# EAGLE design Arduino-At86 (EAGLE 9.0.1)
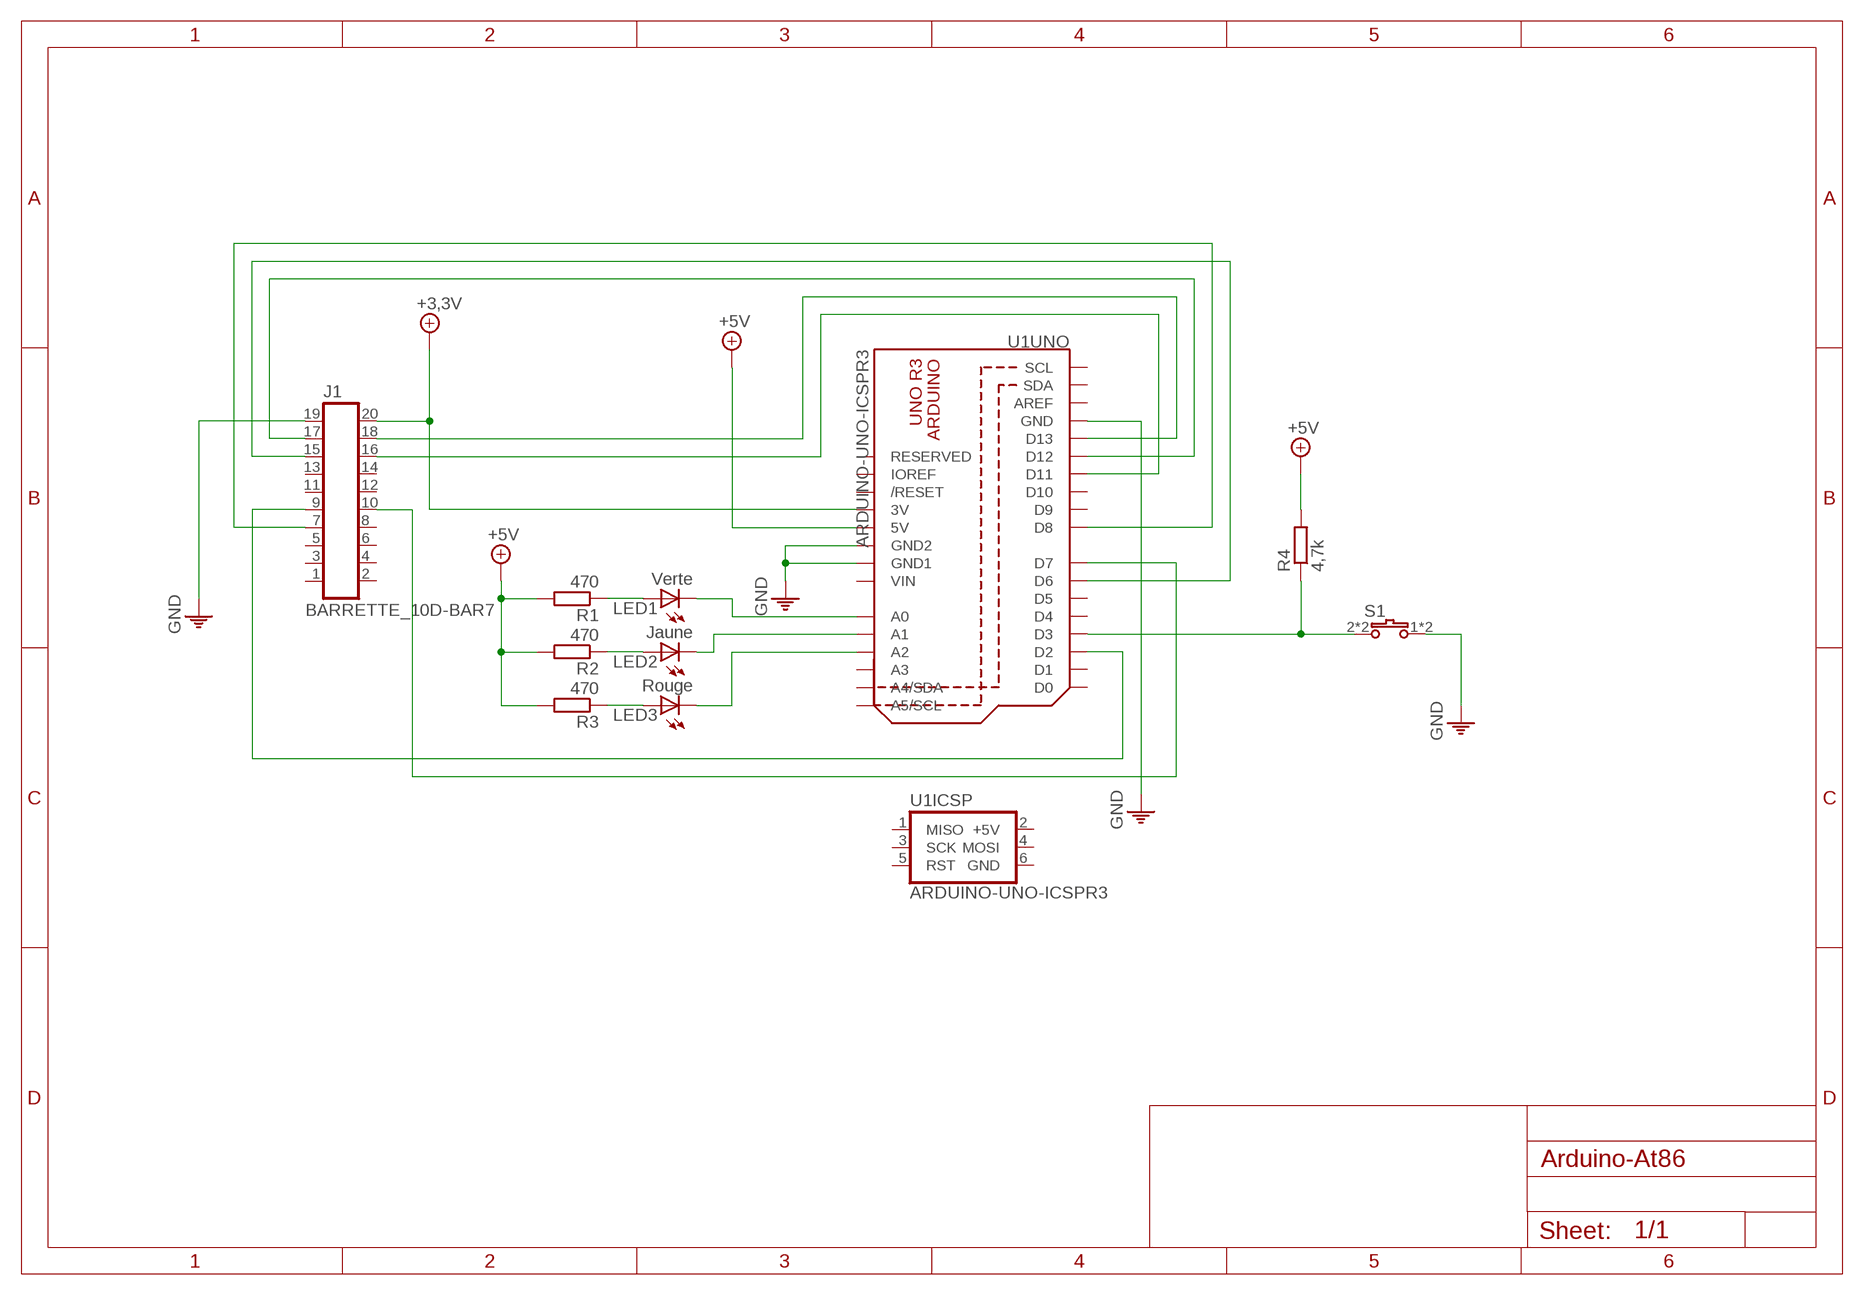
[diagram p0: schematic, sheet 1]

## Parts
J1  BARRETTE_10D-BAR7  [MA010-D]
LED1  Verte  LED3MM  [LED3MM]
LED2  Jaune  LED3MM  [LED3MM]
LED3  Rouge  LED3MM  [LED3MM]
R1  470  RCMS1206  [RCMS1206]
R2  470  RCMS1206  [RCMS1206]
R3  470  RCMS1206  [RCMS1206]
R4  4,7k  RCMS1206  [RCMS1206]
S1  BP-KSA  [TL1105]
U1  ARDUINO-UNO-ICSPR3  [ARD-UNO-ICSP]

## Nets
+3,3V: J1.20 U1.3V(UNO:3V)
+5V: R1.2 R2.2 R3.2 R4.2 U1.5V(UNO:5V)
GND: J1.19 S1.1(S) S1.1@1(S) U1.GND1(UNO:GND1) U1.GND2(UNO:GND2) U1.GND(UNO:GND)
N$1: LED1.A R1.1
N$2: LED2.A R2.1
N$3: LED3.A R3.1
N$4: LED1.K(C) U1.A0(UNO:A0)
N$5: LED2.K(C) U1.A1(UNO:A1)
N$6: R4.1 S1.2(P) S1.2@1(P) U1.D3(UNO:D3)
N$7: LED3.K(C) U1.A2(UNO:A2)
N$8: J1.7 U1.D8(UNO:D8)
N$9: J1.9 U1.D2(UNO:D2)
N$10: J1.15 U1.D6(UNO:D6)
N$11: J1.17 U1.D12(UNO:D12)
N$12: J1.10 U1.D7(UNO:D7)
N$13: J1.18 U1.D13(UNO:D13)
N$14: J1.16 U1.D11(UNO:D11)
Unconnected: J1.1 J1.2 J1.3 J1.4 J1.5 J1.6 J1.8 J1.11 J1.12 J1.13 J1.14 U1.1(ICSP:MISO) U1.3(ICSP:SCK) U1.4(ICSP:MOSI) U1.5(ICSP:RST) U1.A3(UNO:A3) U1.A4(UNO:A4/SDA) U1.A5(UNO:A5/SCL) U1.AREF(UNO:AREF) U1.D0(UNO:D0) U1.D1(UNO:D1) U1.D4(UNO:D4) U1.D5(UNO:D5) U1.D9(UNO:D9) U1.D10(UNO:D10) U1.IOREF(UNO:IOREF) U1.RESERVED(UNO:RESERVED) U1.RESET(UNO:/RESET) U1.SCL(UNO:SCL) U1.SDA(UNO:SDA)

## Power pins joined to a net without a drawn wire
+5V: U1.2(ICSP:+5V)
GND: U1.6(ICSP:GND)
VIN: U1.VIN(UNO:VIN)

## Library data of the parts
J1 = 0IUT xPROJETS:BARRETTE_10D: Barrette Double (2x10 Contacts) GEII/IUT ANGERS; MAGASIN: BARRETTES 7 (Tiroirs n°2-8)
LED1-LED3 = 0IUT OPTO:LED: LED; MAGASIN: LED (Tiroirs n°3-5)
R1-R4 = 0IUT RLCQ:R: Résistance Européenne; MAGASIN: (MAG-CMS)
S1 = 0IUT BP INTER:BP: 1 BP OFF/MOM (Momentané); MAGASIN: BP KSA (Armoire n°6)
U1 = 0IUT DIVERS:ARDUINO-UNO-ICSP: Arduino Uno Avec Connecteur ICSP Doc constructeur GEII/IUT ANGERS

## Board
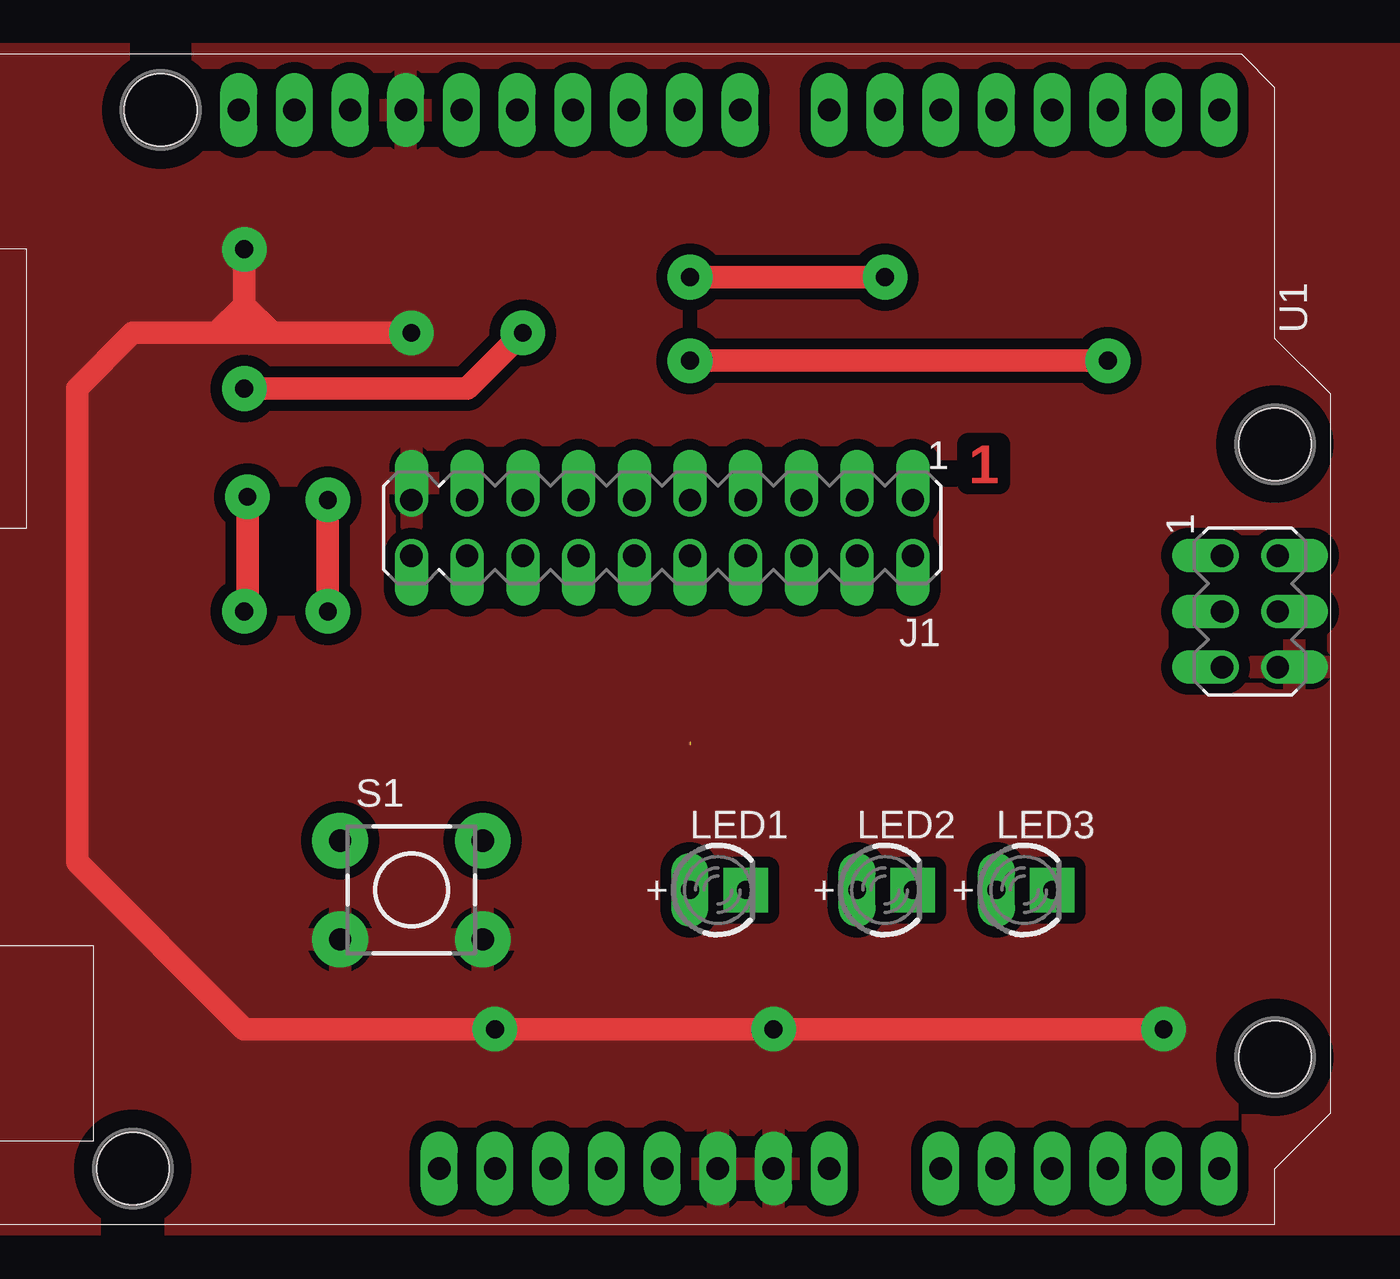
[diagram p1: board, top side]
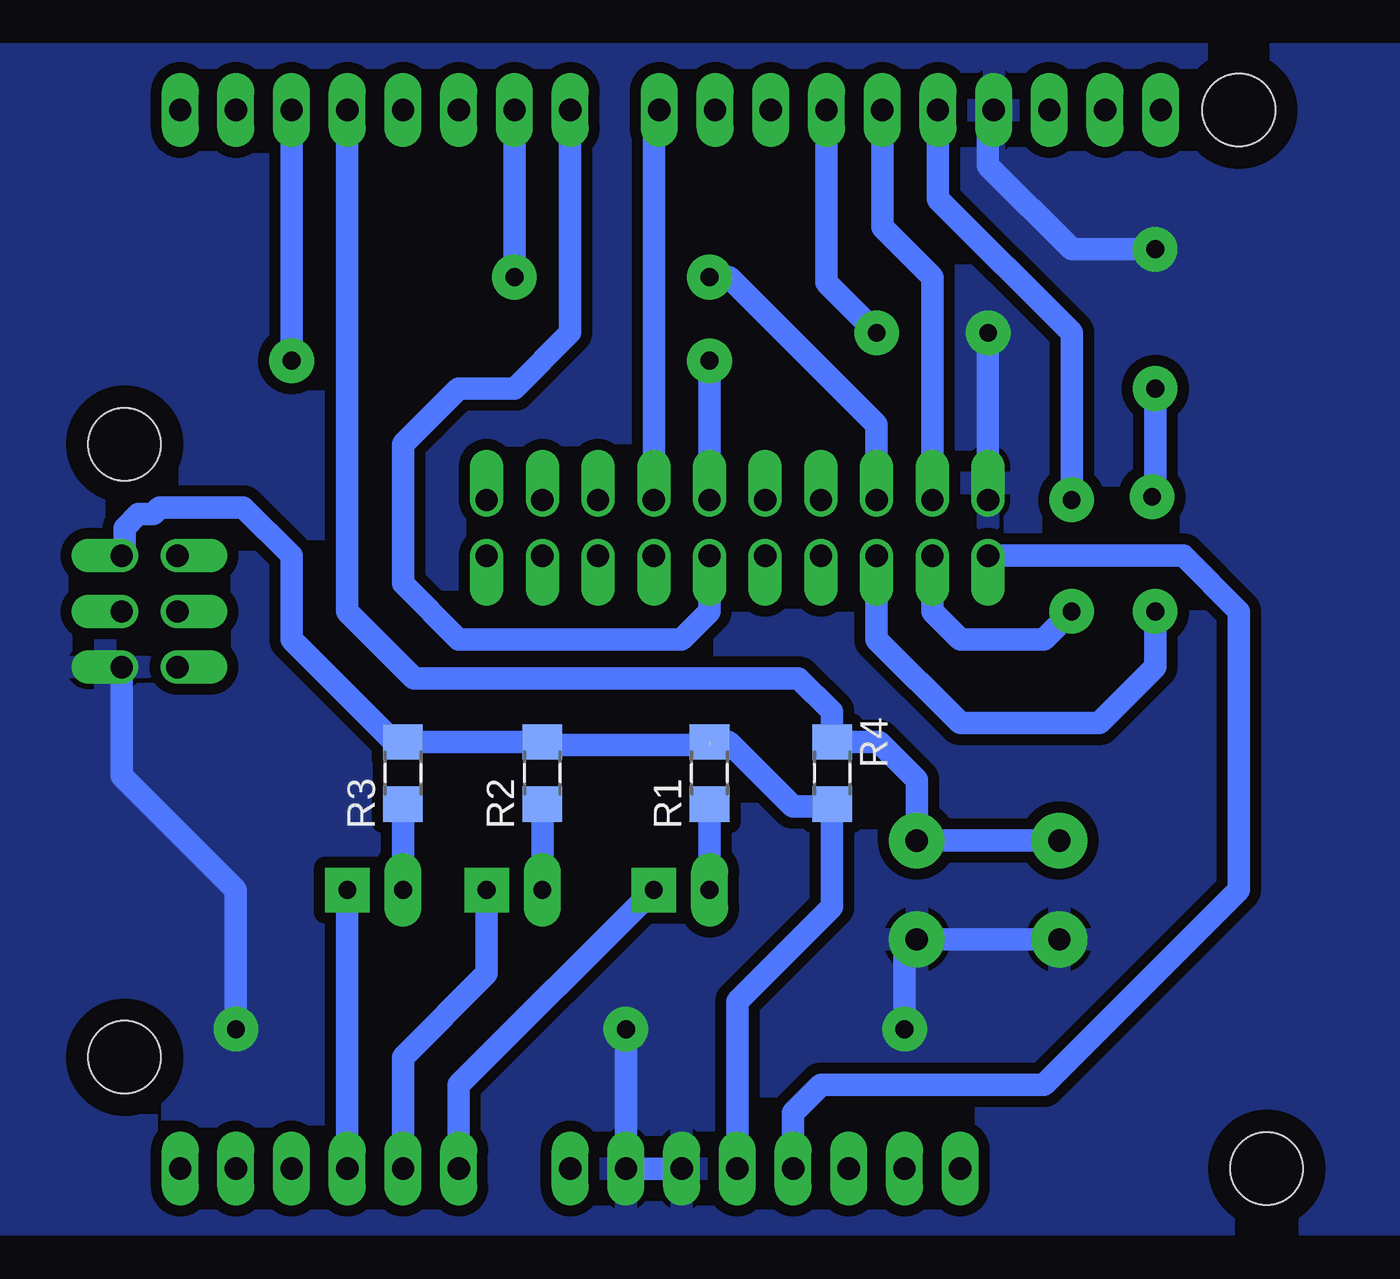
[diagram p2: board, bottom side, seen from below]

No outline drawn. Coordinates in mm, seen from the top.
Copper layers (1*16): Top 0.035mm / dielectric 1.5mm / Bottom 0.035mm
Design rules "default": minimum track width 6mil, minimum drill 0.35mm, track to track 6mil, track to pad 6mil, pad to pad 6mil, via to via 6mil, smd to smd 6mil, copper to edge 40mil, drill to drill 6mil, minimum pad ring 10mil, minimum via ring 8mil, stop-mask expansion 4mil, vias tented up to drill 0mil, thermal gap 10mil

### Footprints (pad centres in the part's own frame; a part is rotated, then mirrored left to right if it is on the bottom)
MA010-D = drill 1.016 pad 1.524 offset: 1 -11.43,-1.27; 2 -11.43,1.27; 3 -8.89,-1.27; 4 -8.89,1.27; 5 -6.35,-1.27; 6 -6.35,1.27; 7 -3.81,-1.27; 8 -3.81,1.27; 9 -1.27,-1.27; 10 -1.27,1.27; 11 1.27,-1.27; 12 1.27,1.27; 13 3.81,-1.27; 14 3.81,1.27; 15 6.35,-1.27; 16 6.35,1.27; 17 8.89,-1.27; 18 8.89,1.27; 19 11.43,-1.27; 20 11.43,1.27
LED3MM = drill 0.813 pad 1.676 long: A -1.27,0 | drill 0.813 pad 2.032 square: K 1.27,0
RCMS1206 = smd 1.6 x 1.803: 1 -1.422,0; 2 1.422,0
TL1105 = drill 1.016 pad 2.54: 1 -3.25,-2.25; 1@1 3.25,-2.25; 2 -3.25,2.25; 2@1 3.25,2.25
ARD-UNO-ICSP = drill 1.016 pad 1.524 offset: 1 28.067,3.81; 2 30.607,3.81; 3 28.067,1.27; 4 30.607,1.27; 5 28.067,-1.27; 6 30.607,-1.27 | drill 1.016 pad 1.676 long: 3V 0,-24.13; 5V 2.54,-24.13; A0 15.24,-24.13; A1 17.78,-24.13; A2 20.32,-24.13; A3 22.86,-24.13; A4 25.4,-24.13; A5 27.94,-24.13; AREF -11.684,24.13; D0 27.94,24.13; D1 25.4,24.13; D2 22.86,24.13; D3 20.32,24.13; D4 17.78,24.13; D5 15.24,24.13; D6 12.7,24.13; D7 10.16,24.13; D8 6.096,24.13; D9 3.556,24.13; D10 1.016,24.13; D11 -1.524,24.13; D12 -4.064,24.13; D13 -6.604,24.13; GND -9.144,24.13; GND1 7.62,-24.13; GND2 5.08,-24.13; IOREF -5.08,-24.13; RESERVED -7.62,-24.13; RESET -2.54,-24.13; SCL -16.764,24.13; SDA -14.224,24.13; VIN 10.16,-24.13 | hole 3.302: -20.32,24.13; 30.48,8.89; 30.48,-19.05; -21.59,-24.13

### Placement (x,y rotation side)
J1  45.72,39.37 180 top
LED1  48.26,22.86 0 top
LED2  55.88,22.86 0 top
LED3  62.23,22.86 0 top
R1  46.99,28.19 90 bottom
R2  54.61,28.19 90 bottom
R3  60.96,28.19 90 bottom
R4  41.4,28.19 270 bottom
S1  34.29,22.86 0 top
U1  43.18,34.29 0 top

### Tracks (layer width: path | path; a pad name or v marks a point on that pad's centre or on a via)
+3,3V
  Bottom 1.016: U1.3V 43.18,12.7 41.91,13.97 31.75,13.97 22.86,22.86 22.86,35.56 25.4,38.1 J1.20
+5V  (1 unrouted)
  Bottom 1.016: 46.99,29.46 54.46,29.46 R2.2 R3.2 61.11,29.36 66.04,34.29 66.04,38.1 68.24,40.3 72.05,40.3 72.34,40.01 73.03,40.01 73.66,39.37 73.66,38.23 U1.2 | U1.5V 45.72,17.78 41.4,22.1 R4.2 41.5,26.67 43.18,26.67 46.13,29.62 R1.2
GND  (via drill 0.81 pad 2.03)
  Top 1.016: v68.58,16.51 v50.8,16.51 v38.1,16.51 26.67,16.51 19.05,24.13 19.05,45.72 21.59,48.26 25.4,48.26 | 25.4,48.26 26.67,48.26 | 26.67,48.26 27.94,48.26 | 27.94,48.26 v34.29,48.26 | v26.67,52.07 26.67,49.53 | 26.67,49.53 26.67,48.26 | 26.67,49.53 25.4,48.26 | 26.67,49.53 27.94,48.26
  Bottom 1.016: S1.1 S1.1@1 38.1,20.05 v38.1,16.51 | U1.GND2 U1.GND1 v50.8,16.51 | v34.29,48.26 J1.19 | v68.58,16.51 68.58,22.86 73.79,28.07 U1.6 | U1.GND 34.29,58.17 34.29,55.88 30.48,52.07 v26.67,52.07
  pour Bottom (isolate 0.508): 7.62,60.96 80.01,60.96 80.01,7.62 7.62,7.62
  pour Top (isolate 0.508): 7.62,60.96 80.01,60.96 80.01,7.62 7.62,7.62
N$1
  Bottom 1.016: LED1.A R1.1
N$2
  Bottom 1.016: LED2.A R2.1
N$3
  Bottom 1.016: LED3.A R3.1
N$4
  Bottom 1.016: U1.A0 58.42,13.97 LED1.K
N$5
  Bottom 1.016: U1.A1 60.96,15.24 57.15,19.05 LED2.K
N$6
  Bottom 1.016: S1.2 S1.2@1 37.54,27.89 39.27,29.62 R4.1 41.4,30.99 42.93,32.51 60.45,32.51 63.5,35.56 U1.D3
N$7
  Bottom 1.016: U1.A2 LED3.K
N$8
  Bottom 1.016: U1.D8 49.53,58.17 J1.7
N$9  (via drill 0.81 pad 2.03)
  Top 1.016: v66.04,46.99 v46.99,46.99
  Bottom 1.016: U1.D2 v66.04,46.99 | v46.99,46.99 J1.9
N$10  (via drill 0.81 pad 2.03)
  Top 1.016: v55.88,50.8 v46.99,50.8
  Bottom 1.016: U1.D6 v55.88,50.8 | J1.15 39.37,44.07 46.1,50.8 v46.99,50.8
N$11
  Bottom 1.016: U1.D12 39.12,53.09 36.83,50.8 J1.17
N$12
  Bottom 1.016: U1.D7 53.34,48.26 55.88,45.72 58.42,45.72 60.96,43.18 60.96,36.83 58.42,34.29 48.26,34.29 46.99,35.56 J1.10
N$13  (via drill 0.81 pad 2.03)
  Top 1.016: v30.48,40.64 v30.48,35.56
  Bottom 1.016: U1.D13 36.58,54.36 30.48,48.26 v30.48,40.64 | J1.18 36.83,35.56 35.56,34.29 31.75,34.29 v30.48,35.56
N$14  (via drill 0.81 pad 2.03)
  Top 1.016: v26.82,40.79 26.82,35.71 v26.67,35.56 | v39.37,48.26 36.83,45.72 v26.67,45.72
  Bottom 1.016: v26.82,40.79 26.67,40.64 v26.67,45.72 | J1.16 39.37,34.29 35.56,30.48 29.21,30.48 26.67,33.02 v26.67,35.56 | U1.D11 41.66,50.55 v39.37,48.26

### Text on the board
Top: 1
